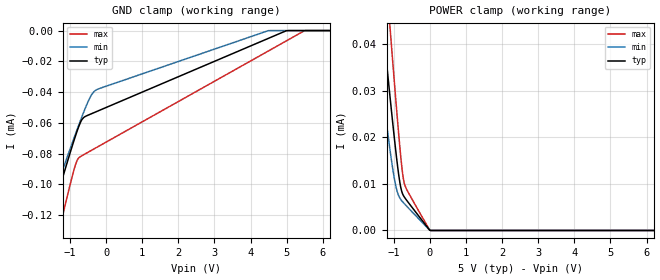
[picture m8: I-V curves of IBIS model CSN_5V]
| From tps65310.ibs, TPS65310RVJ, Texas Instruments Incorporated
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[Model]   CSN_5V
Model_type   Input
Vinl = .8
Vinh = 2.
|   typ   min   max
C_comp   0.01p   0.01p   0.01p
[Voltage Range]   5   4.5   5.5
[Temperature Range]   27   175   -40
[Power Clamp Reference]   5   4.5   5.5
[GND Clamp Reference]   -0   -0   -0
[GND Clamp]
|   Voltage   I(typ)   I(min)   I(max)
-5V       -405.8uA   -352.5uA   -512.2uA
-1.82V    -145.1uA   -132.5uA   -182.9uA
-1.715V   -136.6uA   -125.3uA   -172.1uA
-1.46V    -116.1uA   -108uA     -146.1uA
-1.25V    -99.33uA   -93.83uA   -125uA
-860mV    -69.39uA   -68.05uA   -88.23uA
-695mV    -58.99uA   -57.59uA   -81.76uA
-410mV    -54.15uA   -42.04uA   -77.98uA
-185mV    -51.9uA    -37.71uA   -75.01uA
4.495V    -5.051uA   -18.69nA   -13.26uA
5.485V    0A         0A         -157.7nA
9.985V    0A         0A         0A
[POWER Clamp]
|   Voltage   I(typ)   I(min)   I(max)
-5V       345.6uA    282uA      445.1uA
-1.67V    73.35uA    53.2uA     100.8uA
-1.475V   57.74uA    40.35uA    80.95uA
-1.34V    47.04uA    31.64uA    67.27uA
-1.25V    39.98uA    25.99uA    58.21uA
-1.1V     28.44uA    17.08uA    43.26uA
-965mV    18.55uA    10.4uA     30.13uA
-860mV    11.81uA    7.4uA      20.41uA
-800mV    9.042uA    6.598uA    15.39uA
-725mV    7.394uA    5.902uA    10.73uA
-5mV      58.01nA    59.7nA     106.3nA
9.985V    0A         0A         0A
